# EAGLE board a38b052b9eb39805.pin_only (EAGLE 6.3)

Size 30.35 x 24.13 mm. Coordinates in mm from the lower left corner, seen from the top.
Outline: 0,22.86 arc-90 1.27,24.13 29.08,24.13 arc-90 30.35,22.86 30.35,1.27 arc-90 29.08,0 1.27,0 arc-90 0,1.27 0,22.86
Copper layers (1*16): Top 0.035mm / dielectric 1.5mm / Bottom 0.035mm
Design rules "default *": minimum track width 10mil, minimum drill 20mil, track to track 12mil, track to pad 12mil, pad to pad 10mil, via to via 12mil, smd to smd 0mil, copper to edge 20mil, drill to drill 8mil, minimum pad ring 10mil, minimum via ring 8mil, stop-mask expansion 4mil, vias tented up to drill 20mil, thermal gap 10mil
Holes 3.2 mm at 26.67,21.34 2.67,2.54

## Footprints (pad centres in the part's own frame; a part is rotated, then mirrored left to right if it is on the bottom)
CR1220-THM = drill 2 pad 3.175: +1 -6.604,0; +2 6.604,0 | drill 0.8 pad 3.962 square: - 0,0
C025-025X050 = drill 0.813 pad 1.676 octagon: 1 -1.27,0; 2 1.27,0
DIL08 = drill 0.813 long: 1 -3.81,-3.81; 2 -1.27,-3.81; 3 1.27,-3.81; 4 3.81,-3.81; 5 3.81,3.81; 6 1.27,3.81; 7 -1.27,3.81; 8 -3.81,3.81
1X05 = drill 1.016 long: 1 -5.08,0; 2 -2.54,0; 3 0,0; 4 2.54,0; 5 5.08,0
TC38H = drill 0.813: 1 -1.27,0; 2 1.27,0
0207/10 = drill 0.813 pad 1.676 octagon: 1 -5.08,0; 2 5.08,0

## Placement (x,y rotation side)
BAT  CR1220  [CR1220-THM]  21.97,6.1 180 top
C1  0.1uF  [C025-025X050]  3.56,8.64 180 top
IC3  DS1307  [DIL08]  11.81,18.29 90 top
JP2  [1X05]  2.03,17.14 90 top
Q1  32.768  [TC38H]  18.41,15.75 270 top
R1  2.2k  [0207/10]  11.43,6.6 270 top
R2  2.2K  [0207/10]  8.38,6.6 90 top
U$1  [ADAFRUIT200MIL]  14.48,11.43 180 top

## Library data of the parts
BAT C1 IC3 R1 R2 U$1 = adafruit
JP2 = pinhead
Q1 = crystal

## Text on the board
Top: CC BY-SA
tPlace: GND | DS1307 | RTC | 5V | Breakout | SDA | SCL | SQW | adafruit!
